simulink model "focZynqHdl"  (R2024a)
settings: Solver=FixedStepDiscrete  StartTime=0.0  StopTime=inf  RelTol=1e-3
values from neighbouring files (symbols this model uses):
  dataRange = Rotor velocity
                        radian/sec
                        800.0
                        -800.0
                    
                
                
                    
                        Phase current
                        Ampere
                        12.0
                        -12.0    [focZynqData.sldd]
  encoder = US Digital E2-1250-197-HI
                0.0
                0
                1250.0
                5000.0
                0.0012566370614359172
                0
                20.0    [focZynqData.sldd]
  paramAdcAmperePerCount = -0.000960526315789474 -0.000968421052631579
                
                    
                        Auto
                        
                        
                        -1.0
                        Simulink
                        Parameter
                        Default    [focZynqData.sldd]
  paramAdcCountAtZeroAmpere = 32600.0 32700.0
                
                    
                        Auto
                        
                        
                        -1.0
                        Simulink
                        Parameter
                        Default
                        
                            
                                0    [focZynqData.sldd]
  paramCurrentControlI = 1774.2
                
                    
                        Auto
                        
                        
                        -1.0
                        Simulink
                        Parameter
                        Default
                        
                            
                                0    [focZynqData.sldd]
  paramCurrentControlP = 1.36193
                
                    
                        Auto
                        
                        
                        -1.0
                        Simulink
                        Parameter
                        Default
                        
                            
                                0    [focZynqData.sldd]
  paramCurrentControlSatVoltage = 13.856406460551021
                
                    
                        Auto
                        
                        
                        -1.0
                        Simulink
                        Parameter
                        Default
                        
                            
                                0    [focZynqData.sldd]
  paramEncoderRotorPositionPerCount = 0.0012566370614359172
                
                    
                        Auto
                        
                        
                        -1.0
                        Simulink
                        Parameter
                        Default
                        
                            
                                0    [focZynqData.sldd]
  paramOverCurrentDuration = 0.05
                
                    
                        Auto
                        
                        
                        -1.0
                        Simulink
                        Parameter
                        Default
                        
                            
                                0    [focZynqData.sldd]
  paramOverCurrentEnable = 0.0
                
                    
                        Auto
                        
                        
                        -1.0
                        Simulink
                        Parameter
                        Default
                        
                            
                                0    [focZynqData.sldd]
  paramOverCurrentLimit = 10.45
                
                    
                        Auto
                        
                        
                        -1.0
                        Simulink
                        Parameter
                        Default
                        
                            
                                0    [focZynqData.sldd]
  paramPwmCompareAtZeroVolt = 500.0
                
                    
                        Auto
                        
                        
                        -1.0
                        Simulink
                        Parameter
                        Default
                        
                            
                                0    [focZynqData.sldd]
  paramPwmCompareMax = 1000.0
                
                    
                        Auto
                        
                        
                        -1.0
                        Simulink
                        Parameter
                        Default
                        
                            
                                0    [focZynqData.sldd]
  paramPwmComparePerVolt = 41.666666666666664
                
                    
                        Auto
                        
                        
                        -1.0
                        Simulink
                        Parameter
                        Default
                        
                            
                                0    [focZynqData.sldd]
  pmsm = Dyno 1: BLY172D-24V-4000 Anaheim Automation
                BLY172D-24V-4000 Anaheim Automation
Phase A leads B leads C for counterclockwise rotation
-----------------------------------------------------
Phase A = Yellow
Phase B = Red
Phase C = Black
                
                    
                        Watt
                        Volt
                        rad/sec    [focZynqData.sldd]
  pwm = 2.0E-8
                4.0E-5
                1000.0
                2000.0
                5.0
                1.0E-7    [focZynqData.sldd]
  sampleTime = 4.0E-5
                0.001
                0.001
                4.0E-5
                2.0E-8
                4.0E-5
                0.001
                2.0E-8
                2.0E-8
                2.0E-8    [focZynqData.sldd]
undefined symbols (not defined in the file or in its folder): hex2dec
libraries: simulink x8
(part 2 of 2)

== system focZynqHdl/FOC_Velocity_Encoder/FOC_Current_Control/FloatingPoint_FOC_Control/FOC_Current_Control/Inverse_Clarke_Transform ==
  note: Inverse Clarke Transform
  note: Converts direct axis (alpha) component and the quadrature axis (beta) component to balanced three-phase quantities The alpha and beta components are dependent on time and speed.
  Alpha : Inport
  Beta : Inport  Port=2
  Add : Sum  Inputs=-+  OutDataTypeStr=Inherit: Inherit via back propagation
  Add1 : Sum  Inputs=--  OutDataTypeStr=Inherit: Inherit via back propagation
  Data_Type_Convert : DataTypeConversion  RndMeth=Simplest
  Gain : Gain  Gain=1/2  OutDataTypeStr=Inherit: Inherit via back propagation
  Gain1 : Gain  Gain=sqrt(3)/2  OutDataTypeStr=Inherit: Inherit via back propagation
  Mux : Mux  Inputs=3
  ABC : Outport  VectorParamsAs1DForOutWhenUnconnected=off
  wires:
  Gain/1 -> Add1/1, Add/1
  Gain1/1 -> Add1/2, Add/2
  Add/1 -> Mux/2
  Add1/1 -> Mux/3
  Beta/1 -> Gain1/1
  Alpha/1 -> Gain/1, Data_Type_Convert/1
  Mux/1 -> ABC/1
  Data_Type_Convert/1 -> Mux/1

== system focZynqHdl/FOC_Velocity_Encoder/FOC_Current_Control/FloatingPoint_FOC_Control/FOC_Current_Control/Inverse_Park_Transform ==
  note: Inverse Park Transform
  note: Converts orthogonal rotating reference frame (dq) to two-phase orthogonal stationary reference frame (alpha, beta)
  D : Inport
  Q : Inport  Port=2
  Sin_Coefficient : Inport  Port=3
  Cos_Coefficient : Inport  Port=4
  Add1 : Sum  Inputs=+-  OutDataTypeStr=Inherit: Inherit via back propagation
  Add2 : Sum  OutDataTypeStr=Inherit: Inherit via back propagation
  Cos_Coefficient1 : InportShadow  Port=4
  Product{1..4} (4 alike) : Product  OutDataTypeStr=Inherit: Inherit via back propagation  RndMeth=Simplest
  Sin_Coefficient1 : InportShadow  Port=3
  Alpha : Outport  VectorParamsAs1DForOutWhenUnconnected=off
  Beta : Outport  Port=2  VectorParamsAs1DForOutWhenUnconnected=off
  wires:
  Add2/1 -> Beta/1
  Add1/1 -> Alpha/1
  Product3/1 -> Add2/1
  Product4/1 -> Add2/2
  Product1/1 -> Add1/1
  Product2/1 -> Add1/2
  Cos_Coefficient1/1 -> Product4/2
  Sin_Coefficient/1 -> Product2/2
  D/1 -> Product3/1, Product1/1
  Q/1 -> Product2/1, Product4/1
  Sin_Coefficient1/1 -> Product3/2
  Cos_Coefficient/1 -> Product1/2

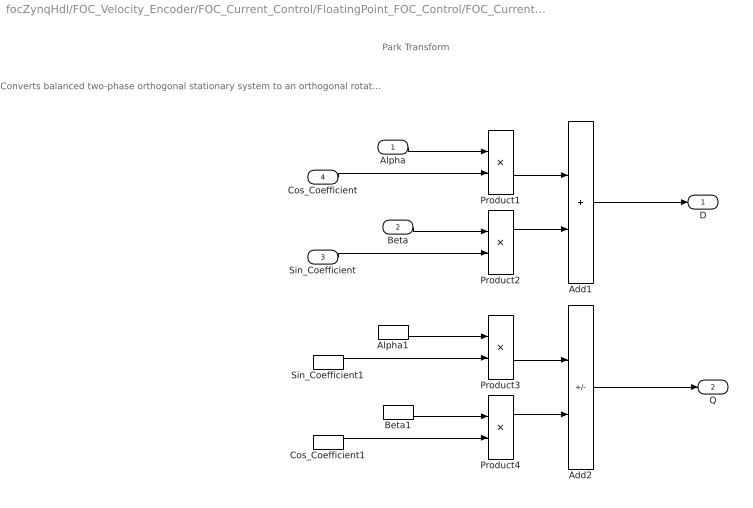
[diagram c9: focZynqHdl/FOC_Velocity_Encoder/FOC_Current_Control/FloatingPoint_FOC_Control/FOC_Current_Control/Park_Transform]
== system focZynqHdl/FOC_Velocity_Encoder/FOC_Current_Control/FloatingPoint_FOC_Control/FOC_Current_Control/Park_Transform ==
  note: Park Transform
  note: Converts balanced two-phase orthogonal stationary system to an orthogonal rotating reference frame.
  Alpha : Inport
  Beta : Inport  Port=2
  Sin_Coefficient : Inport  Port=3
  Cos_Coefficient : Inport  Port=4
  Add1 : Sum  OutDataTypeStr=Inherit: Inherit via back propagation
  Add2 : Sum  Inputs=-+  OutDataTypeStr=Inherit: Inherit via back propagation
  Alpha1 : InportShadow
  Beta1 : InportShadow  Port=2
  Cos_Coefficient1 : InportShadow  Port=4
  Product{1..4} (4 alike) : Product  OutDataTypeStr=Inherit: Inherit via back propagation  RndMeth=Simplest
  Sin_Coefficient1 : InportShadow  Port=3
  D : Outport  VectorParamsAs1DForOutWhenUnconnected=off
  Q : Outport  Port=2  VectorParamsAs1DForOutWhenUnconnected=off
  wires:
  Product3/1 -> Add2/1
  Product4/1 -> Add2/2
  Product1/1 -> Add1/1
  Product2/1 -> Add1/2
  Alpha1/1 -> Product3/1
  Sin_Coefficient1/1 -> Product3/2
  Cos_Coefficient1/1 -> Product4/2
  Beta1/1 -> Product4/1
  Alpha/1 -> Product1/1
  Cos_Coefficient/1 -> Product1/2
  Beta/1 -> Product2/1
  Sin_Coefficient/1 -> Product2/2
  Add1/1 -> D/1
  Add2/1 -> Q/1

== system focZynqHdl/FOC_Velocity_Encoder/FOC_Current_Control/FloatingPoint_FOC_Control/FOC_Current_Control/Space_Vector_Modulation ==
  note: Space Vector Modulation
  ABC : Inport
  Add : Sum  OutDataTypeStr=Inherit: Inherit via back propagation
  Add1 : Sum  Inputs=+-  OutDataTypeStr=Inherit: Inherit via back propagation
  Gain : Gain  Gain=0.5  OutDataTypeStr=Inherit: Inherit via back propagation
  Max : MinMax  Function=max
  Min : MinMax
  ABC_SVM : Outport  VectorParamsAs1DForOutWhenUnconnected=off
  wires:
  Add/1 -> Gain/1
  Max/1 -> Add/1
  Min/1 -> Add/2
  Gain/1 -> Add1/2
  ABC/1 -> Add1/1, Max/1, Min/1
  Add1/1 -> ABC_SVM/1

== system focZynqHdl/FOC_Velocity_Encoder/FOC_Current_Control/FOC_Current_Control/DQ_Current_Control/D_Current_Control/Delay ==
  note: Delay With Reset
  In : Inport
  Reset : Inport  Port=2
  Constant : Constant  Value=0  OutDataTypeStr=Inherit: Inherit via back propagation  SampleTime=-1
  Delay1 : Delay  DelayLength=1
  Reset1 : InportShadow  Port=2
  Switch : Switch  Criteria=u2 ~= 0
  Switch1 : Switch  Criteria=u2 ~= 0
  Out : Outport  VectorParamsAs1DForOutWhenUnconnected=off
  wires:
  In/1 -> Switch1/3
  Reset/1 -> Switch1/2
  Reset1/1 -> Switch/2
  Constant/1 -> Switch/1, Switch1/1
  Switch1/1 -> Delay1/1
  Switch/1 -> Out/1
  Delay1/1 -> Switch/3

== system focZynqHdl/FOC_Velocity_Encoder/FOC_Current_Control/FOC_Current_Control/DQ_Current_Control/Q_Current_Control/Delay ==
  note: Delay With Reset
  In : Inport
  Reset : Inport  Port=2
  Constant : Constant  Value=0  OutDataTypeStr=Inherit: Inherit via back propagation  SampleTime=-1
  Delay1 : Delay  DelayLength=1
  Reset1 : InportShadow  Port=2
  Switch : Switch  Criteria=u2 ~= 0
  Switch1 : Switch  Criteria=u2 ~= 0
  Out : Outport  VectorParamsAs1DForOutWhenUnconnected=off
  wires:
  In/1 -> Switch1/3
  Reset/1 -> Switch1/2
  Reset1/1 -> Switch/2
  Constant/1 -> Switch/1, Switch1/1
  Switch1/1 -> Delay1/1
  Switch/1 -> Out/1
  Delay1/1 -> Switch/3

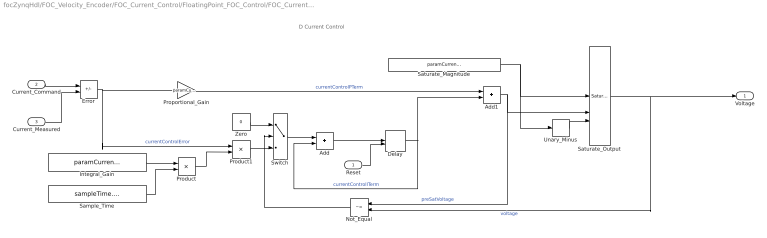
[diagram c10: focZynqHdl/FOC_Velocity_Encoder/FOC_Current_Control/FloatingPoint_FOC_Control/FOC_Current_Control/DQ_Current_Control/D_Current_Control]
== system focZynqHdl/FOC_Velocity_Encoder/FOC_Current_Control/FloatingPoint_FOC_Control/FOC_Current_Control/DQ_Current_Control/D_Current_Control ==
  note: D Current Control
  Reset : Inport
  Current_Command : Inport  Port=2
  Current_Measured : Inport  Port=3
  Add : Sum  OutDataTypeStr=Inherit: Inherit via back propagation
  Add1 : Sum  OutDataTypeStr=Inherit: Inherit via back propagation
  Delay : Delay  DelayLength=1  ExternalReset=Level
  Error : Sum  Inputs=+-  OutDataTypeStr=Inherit: Inherit via back propagation
  Integral_Gain : Constant  Value=paramCurrentControlI  OutDataTypeStr=Inherit: Inherit via back propagation  SampleTime=-1
  Not_Equal : RelationalOperator  Operator=~=  OutDataTypeStr=boolean
  Product : Product  OutDataTypeStr=Inherit: Inherit via back propagation
  Product1 : Product  OutDataTypeStr=Inherit: Inherit via back propagation
  Proportional_Gain : Gain  Gain=paramCurrentControlP  OutDataTypeStr=Inherit: Inherit via back propagation
  Sample_Time : Constant  Value=sampleTime.CurrentControl  OutDataTypeStr=Inherit: Inherit via back propagation  SampleTime=-1
  Saturate_Magnitude : Constant  Value=paramCurrentControlSatVoltage  OutDataTypeStr=Inherit: Inherit via back propagation  SampleTime=-1
  Saturate_Output : simulink/Discontinuities/Saturation Dynamic  OutMin=[]  OutMax=[]  OutDataTypeStr=Inherit: Same as second input  OutDataType=fixdt(1, 16)  OutScaling=2^-10  DoSatur=off
  Switch : Switch  Criteria=u2 ~= 0  OutDataTypeStr=Inherit: Inherit via back propagation
  Unary_Minus : UnaryMinus
  Zero : Constant  Value=0  OutDataTypeStr=Inherit: Inherit via back propagation  SampleTime=-1
  Voltage : Outport  VectorParamsAs1DForOutWhenUnconnected=off
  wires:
  Product1/1 -> Switch/3
  Product/1 -> Product1/2
  Sample_Time/1 -> Product/2
  Integral_Gain/1 -> Product/1
  Unary_Minus/1 -> Saturate_Output/3
  Saturate_Magnitude/1 -> Unary_Minus/1, Saturate_Output/1
  Add/1 -> Delay/1
  Zero/1 -> Switch/1
  Switch/1 -> Add/1
  Not_Equal/1 -> Switch/2
  Saturate_Output/1 -> Voltage/1, Not_Equal/2  "voltage"
  Error/1 -> Product1/1, Proportional_Gain/1  "currentControlError"
  Proportional_Gain/1 -> Add1/1  "currentControlPTerm"
  Current_Command/1 -> Error/1
  Add1/1 -> Saturate_Output/2, Not_Equal/1  "preSatVoltage"
  Delay/1 -> Add1/2, Add/2  "currentControlITerm"
  Current_Measured/1 -> Error/2
  Reset/1 -> Delay/2

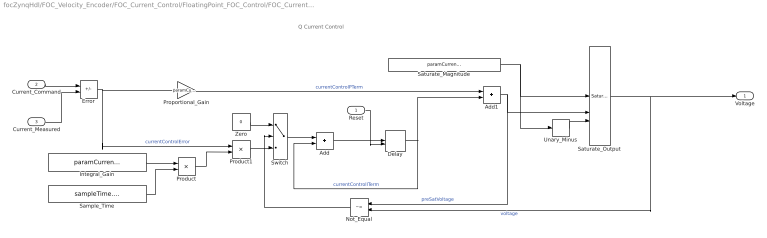
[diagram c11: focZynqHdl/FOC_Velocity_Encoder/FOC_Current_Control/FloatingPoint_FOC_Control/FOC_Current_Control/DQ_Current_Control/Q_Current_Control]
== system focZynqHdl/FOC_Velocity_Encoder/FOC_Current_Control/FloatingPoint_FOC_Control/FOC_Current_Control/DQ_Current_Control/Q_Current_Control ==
  note: Q Current Control
  Reset : Inport
  Current_Command : Inport  Port=2
  Current_Measured : Inport  Port=3
  Add : Sum  OutDataTypeStr=Inherit: Inherit via back propagation
  Add1 : Sum  OutDataTypeStr=Inherit: Inherit via back propagation
  Delay : Delay  DelayLength=1  ExternalReset=Level
  Error : Sum  Inputs=+-  OutDataTypeStr=Inherit: Inherit via back propagation
  Integral_Gain : Constant  Value=paramCurrentControlI  OutDataTypeStr=Inherit: Inherit via back propagation  SampleTime=-1
  Not_Equal : RelationalOperator  Operator=~=  OutDataTypeStr=boolean
  Product : Product  OutDataTypeStr=Inherit: Inherit via back propagation
  Product1 : Product  OutDataTypeStr=Inherit: Inherit via back propagation
  Proportional_Gain : Gain  Gain=paramCurrentControlP  OutDataTypeStr=Inherit: Inherit via back propagation
  Sample_Time : Constant  Value=sampleTime.CurrentControl  OutDataTypeStr=Inherit: Inherit via back propagation  SampleTime=-1
  Saturate_Magnitude : Constant  Value=paramCurrentControlSatVoltage  OutDataTypeStr=Inherit: Inherit via back propagation  SampleTime=-1
  Saturate_Output : simulink/Discontinuities/Saturation Dynamic  OutMin=[]  OutMax=[]  OutDataTypeStr=Inherit: Same as second input  OutDataType=fixdt(1, 16)  OutScaling=2^-10  DoSatur=off
  Switch : Switch  Criteria=u2 ~= 0  OutDataTypeStr=Inherit: Inherit via back propagation
  Unary_Minus : UnaryMinus
  Zero : Constant  Value=0  OutDataTypeStr=Inherit: Inherit via back propagation  SampleTime=-1
  Voltage : Outport  VectorParamsAs1DForOutWhenUnconnected=off
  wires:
  Product1/1 -> Switch/3
  Product/1 -> Product1/2
  Sample_Time/1 -> Product/2
  Integral_Gain/1 -> Product/1
  Unary_Minus/1 -> Saturate_Output/3
  Saturate_Magnitude/1 -> Unary_Minus/1, Saturate_Output/1
  Add/1 -> Delay/1
  Zero/1 -> Switch/1
  Switch/1 -> Add/1
  Not_Equal/1 -> Switch/2
  Saturate_Output/1 -> Voltage/1, Not_Equal/2  "voltage"
  Error/1 -> Product1/1, Proportional_Gain/1  "currentControlError"
  Proportional_Gain/1 -> Add1/1  "currentControlPTerm"
  Current_Command/1 -> Error/1
  Add1/1 -> Saturate_Output/2, Not_Equal/1  "preSatVoltage"
  Delay/1 -> Add1/2, Add/2  "currentControlITerm"
  Current_Measured/1 -> Error/2
  Reset/1 -> Delay/2

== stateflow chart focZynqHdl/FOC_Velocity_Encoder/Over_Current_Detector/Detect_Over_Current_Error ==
  state Detect Over Current Error [group]
  state If either Phase A Current (current[0]) or Phase B Current are above the threshold for a given duration, generate an error. [group]
    The error is reset when over current detection is disabled.
  state No_Error
    entry: error = false;
  state Possible_Error
  state Wait_For_Reset
  state Error
    entry: error = true;
  (default) -> No_Error
  No_Error -> Possible_Error : [enableOverCurrentDetect && ...  ((phaseCurrentA >= overCurrentLimit) || ...   (phaseCurrentB >= overCurrentLimit)    ) ]
  Possible_Error -> No_Error : [(phaseCurrentA < overCurrentLimit) && ...  (phaseCurrentB< overCurrentLimit)]
  Wait_For_Reset -> No_Error : [enableOverCurrentDetect]
  Possible_Error -> Error : [after(overCurrentDurationTicks,tick)]
  Error -> Wait_For_Reset : [~enableOverCurrentDetect]
  data: enableOverCurrentDetect input; phaseCurrentA input; phaseCurrentB input; overCurrentLimit input; overCurrentDurationTicks input; error output boolean

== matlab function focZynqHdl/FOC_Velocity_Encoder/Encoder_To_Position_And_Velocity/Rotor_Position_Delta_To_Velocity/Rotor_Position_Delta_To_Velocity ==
function rotorVelocity = fcn(...                        %#codegen
                          positionDelta,...             % Input
                          positionDeltaBufferLength,... % Constant parameter
                          sampleFrequency)              % Constant parameter
% Copyright 2014 The MathWorks, Inc.

%% States
persistent positionDeltaBuffer;
persistent bufferIndex;

%% Constraints
%  Design maximums used for scaling fixed-point signals
%    sampleFrequency   = 50000 Hz
%    rotorVelocity     = 800 rad/sec
%    deltaSumFrequency = sampleFrequency/positionDeltaBufferLength = 2000 Hz
%    positionDeltaSum  = 6.2832 rad

% Assertions
assert(log2(double(positionDeltaBufferLength)) == floor(double(log2(positionDeltaBufferLength))),...
    'Delay buffer must be a power of two.');

assert(sampleFrequency < 50000,...
    'sampleFrequency must be less than 50000');

assert(sampleFrequency/positionDeltaBufferLength < 2000,...
    'Ratio of sampleFrequency to positionDeltaBufferLength is too large');

% Input data types
positionDelta             = fi(positionDelta,   true,16,12);
sampleFrequency           = fi(sampleFrequency, true,16,-1);
positionDeltaBufferLength = double(positionDeltaBufferLength);
% NOTE: positionDeltaBufferLength is used by intermediate variables and
%       does not introduce double precision data into generated code

% Intermediate variable data types
bufferIndexBitMask       = int32(0);
reciprocalOfBufferLength = fi(1, true,16,14);
positionDeltaSum         = fi(1, true,16,12);
deltaSumFrequency        = fi(1, true,16,4);

% Output data types
rotorVelocity            = fi(1, true,16,5 );

%% Initialize states
if isempty(positionDeltaBuffer)
    positionDeltaBuffer = ...
           zeros(positionDeltaBufferLength,1,...
                 'like', positionDelta);
    bufferIndex = int32(0);
end

%% Initialize constants
bufferIndexBitMask(:) = positionDeltaBufferLength - 1;
reciprocalOfBufferLength(:) = 1/positionDeltaBufferLength;

%% Step 
% Update delay buffer and index (MATLAB is one based indexing)
bufferIndex = bitand(bufferIndex+1, bufferIndexBitMask);
positionDeltaBuffer(bufferIndex+1) = positionDelta;

% Calculate velocity
positionDeltaSum(:) = sum(positionDeltaBuffer);
deltaSumFrequency(:) = sampleFrequency * reciprocalOfBufferLength;
rotorVelocity(:) = positionDeltaSum * deltaSumFrequency;
